(* Logix 5000 AddOnInstructionDefinition export; software revision 16.04 *)

ADD_ON_INSTRUCTION AMCI_ANG1E_Home_CCW   (* revision 1.1, vendor AMCI, ExecuteEnableInFalse *)
// Revision note:
// Version 1.1 added the slot_axis number and the input parameters can now be tags or discrete values.
VAR_INPUT
   Axis_Status_Bits : INT; {required}
   slot_axis_number : INT; {required}
   Type_0_for_standard_1_for_indexed : BOOL;
   Programmed_Speed : DINT; {required}
   Acceleration : INT; {required}
   Deceleration : INT; {required}
   jerk : INT;
END_VAR
VAR_IN_OUT
   AMCI_ANG1E_output_data : INT[10]; {required}
END_VAR
VAR_OUTPUT
   EN : BOOL; {visible}
   ER : BOOL; {visible}
END_VAR
VAR
   Upper_Result_X_1000 : DINT;
   command_data_block : INT[10];
        [0]   // Command Bits MSW
        [1]   // Command Bits LSW
        [2]   // Upper Target Position
        [3]   // Lower Target Position
        [4]   // Upper Programmed Speed
        [5]   // Lower Programmed Speed
   index : INT;
END_VAR

ROUTINE EnableInFalse   (* ladder *)
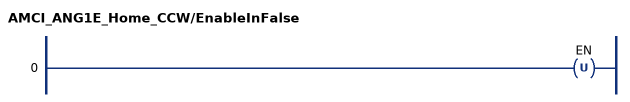
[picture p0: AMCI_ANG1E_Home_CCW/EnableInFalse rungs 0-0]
   0: OTU(EN);
END_ROUTINE

ROUTINE Logic   (* ladder *)
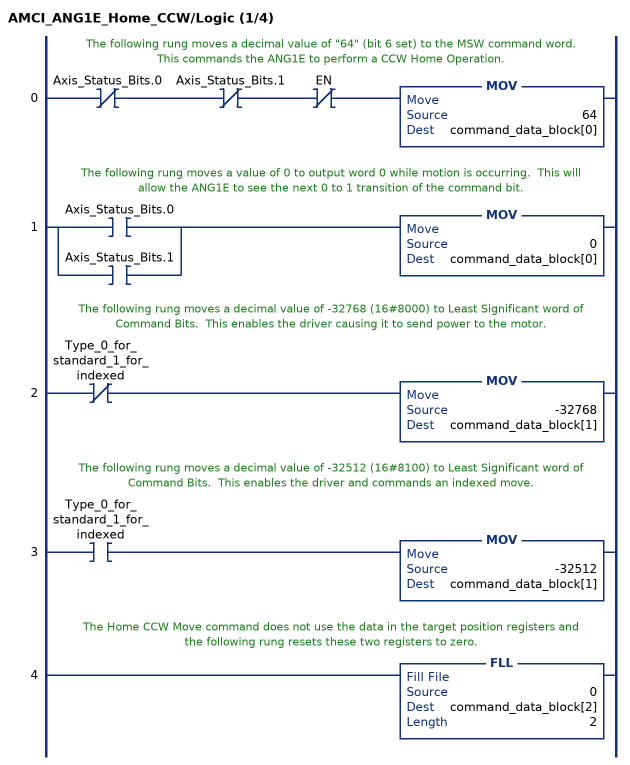
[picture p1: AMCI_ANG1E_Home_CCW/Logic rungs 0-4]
   // The following rung moves a decimal value of "64" (bit 6 set) to the MSW command word.  This commands the ANG1E to perform a CCW Home Operation.
   0: XIO(Axis_Status_Bits.0)XIO(Axis_Status_Bits.1)XIO(EN)MOV(64,command_data_block[0]);
   // The following rung moves a value of 0 to output word 0 while motion is occurring.  This will allow the ANG1E to see the next 0 to 1 transition of the command bit.
   1: [XIC(Axis_Status_Bits.0) ,XIC(Axis_Status_Bits.1) ]MOV(0,command_data_block[0]);
   // The following rung moves a decimal value of -32768 (16#8000) to Least Significant word of Command Bits.  This enables the driver causing it to send power to the motor.
   2: XIO(Type_0_for_standard_1_for_indexed)MOV(-32768,command_data_block[1]);
   // The following rung moves a decimal value of -32512 (16#8100) to Least Significant word of Command Bits.  This enables the driver and commands an indexed move.
   3: XIC(Type_0_for_standard_1_for_indexed)MOV(-32512,command_data_block[1]);
   // The Home CCW Move command does not use the data in the target position registers and the following rung resets these two registers to zero.
   4: FLL(0,command_data_block[2],2);
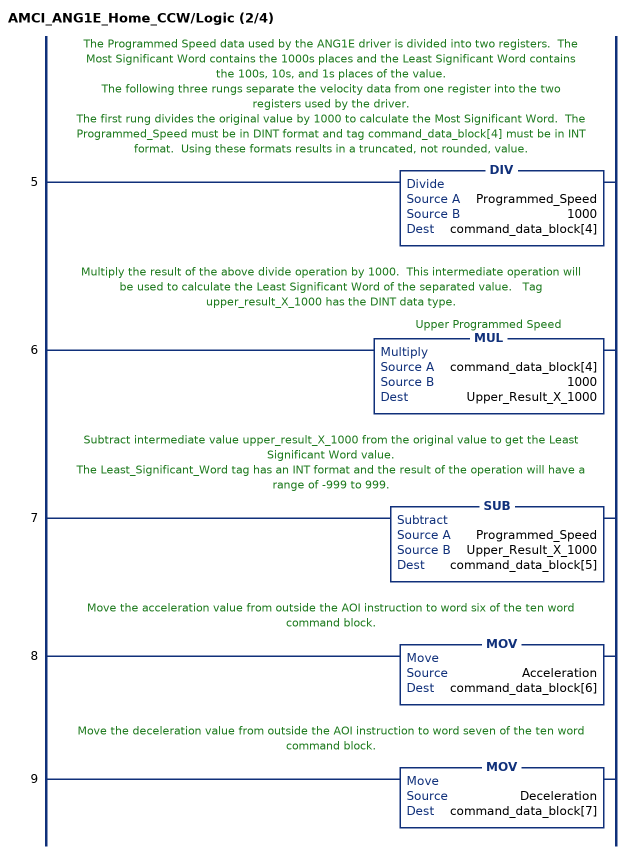
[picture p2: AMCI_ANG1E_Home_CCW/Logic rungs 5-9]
   // The Programmed Speed data used by the ANG1E driver is divided into two registers.  The Most Significant Word contains the 1000s places and the Least Significant Word contains the 100s, 10s, and 1s places of the value.
   // The following three rungs separate the velocity data from one register into the two registers used by the driver.
   // The first rung divides the original value by 1000 to calculate the Most Significant Word.  The Programmed_Speed must be in DINT format and tag command_data_block[4] must be in INT format.  Using these formats results in a truncated, not rounded, value.
   5: DIV(Programmed_Speed,1000,command_data_block[4]);
   // Multiply the result of the above divide operation by 1000.  This intermediate operation will be used to calculate the Least Significant Word of the separated value.   Tag upper_result_X_1000 has the DINT data type.
   6: MUL(command_data_block[4],1000,Upper_Result_X_1000);
   // Subtract intermediate value upper_result_X_1000 from the original value to get the Least Significant Word value.
   // The Least_Significant_Word tag has an INT format and the result of the operation will have a range of -999 to 999.
   7: SUB(Programmed_Speed,Upper_Result_X_1000,command_data_block[5]);
   // Move the acceleration value from outside the AOI instruction to word six of the ten word command block.
   8: MOV(Acceleration,command_data_block[6]);
   // Move the deceleration value from outside the AOI instruction to word seven of the ten word command block.
   9: MOV(Deceleration,command_data_block[7]);
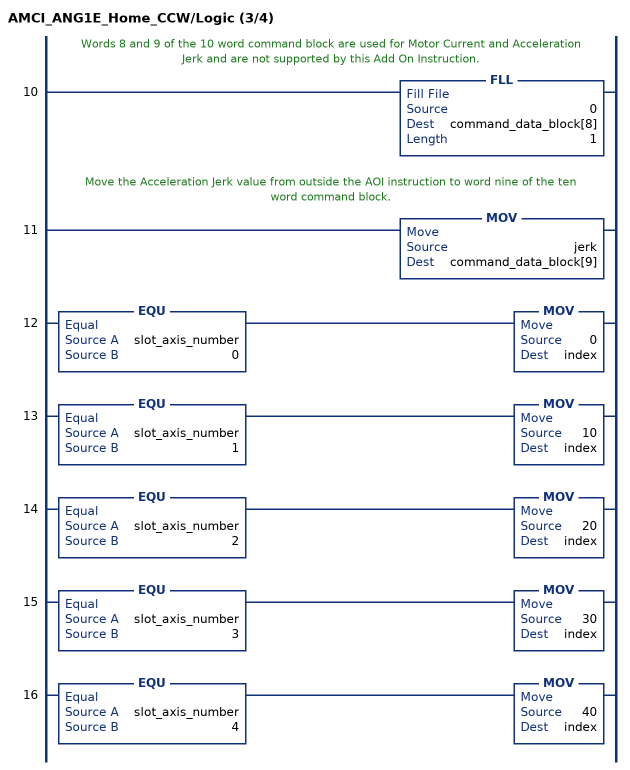
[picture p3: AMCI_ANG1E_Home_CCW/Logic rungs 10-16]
   // Words 8 and 9 of the 10 word command block are used for Motor Current and Acceleration Jerk and are not supported by this Add On Instruction.
   10: FLL(0,command_data_block[8],1);
   // Move the Acceleration Jerk value from outside the AOI instruction to word nine of the ten word command block.
   11: MOV(jerk,command_data_block[9]);
   12: EQU(slot_axis_number,0)MOV(0,index);
   13: EQU(slot_axis_number,1)MOV(10,index);
   14: EQU(slot_axis_number,2)MOV(20,index);
   15: EQU(slot_axis_number,3)MOV(30,index);
   16: EQU(slot_axis_number,4)MOV(40,index);
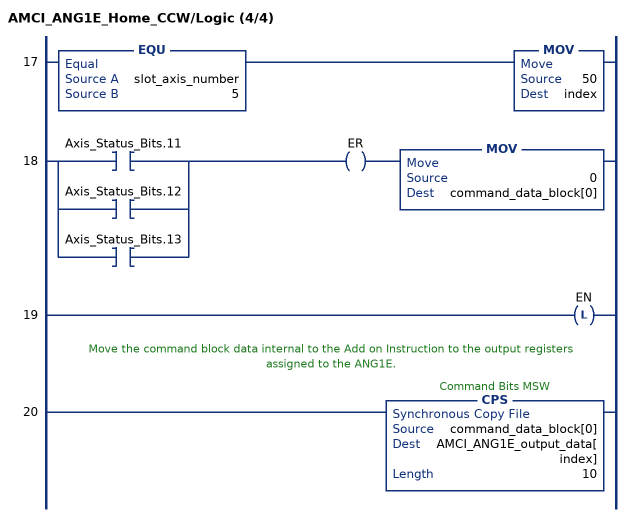
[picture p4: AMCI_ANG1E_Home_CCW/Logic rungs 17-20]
   17: EQU(slot_axis_number,5)MOV(50,index);
   18: [XIC(Axis_Status_Bits.11) ,XIC(Axis_Status_Bits.12) ,XIC(Axis_Status_Bits.13) ]OTE(ER)MOV(0,command_data_block[0]);
   19: OTL(EN);
   // Move the command block data internal to the Add on Instruction to the output registers assigned to the ANG1E.
   20: CPS(command_data_block[0],AMCI_ANG1E_output_data[index],10);
END_ROUTINE
END_ADD_ON_INSTRUCTION
